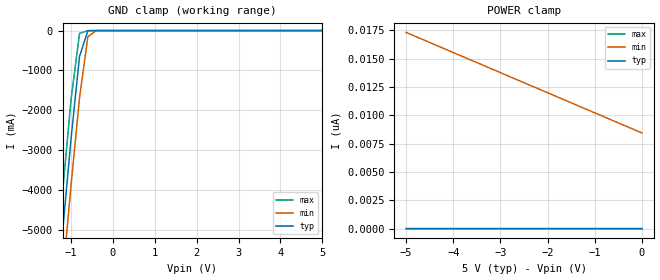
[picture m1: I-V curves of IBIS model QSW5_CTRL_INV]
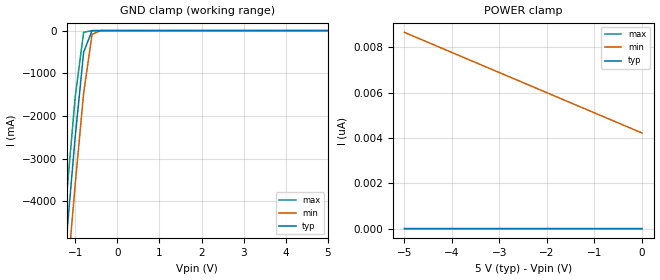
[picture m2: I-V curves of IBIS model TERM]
| I/O Buffer Information Specification (IBIS) Version 3.2 (August 20, 1999)
| IBIS is a standard for electronic behavioral specifications of integrated
| circuit input/output analog characteristics.
[IBIS Ver]   3.2
[File Name]   qs3384.ibs
[File Rev]   2.0
[Date]   Wednesday, June 9, 2004
[Source]   Integrated Device Technology, Inc.
[Notes]   1.Temperatures: typ=25C, min=-40C, max=100C
[Disclaimer]
Integrated Device Technology, Inc. ("IDT") hereby grants the user of this
IBIS model ("User") a non-exclusive, nontransferable license to use this
IBIS model under the following terms: The User is granted this license only
to use the IBIS model for demonstration purposes only and is not granted
rights to sell, copy (except as needed to run the IBIS model), rent, lease
or sub-license (except for demonstration) the IBIS model in whole or in
part, or in modified form to anyone. The User may modify the IBIS model to
suit its specific applications, but  rights to derivative works and such
modifications shall belong to IDT.
THIS IBIS MODEL IS PROVIDED ON AN AS IS" BASIS AND IDT  MAKES ABSOLUTELY NO
WARRANTY WITH RESPECT TO THE INFORMATION CONTAINED HEREIN.  IDT DISCLAIMS
AND USER WAIVES ALL WARRANTIES, EXPRESS AND IMPLIED, INCLUDING WARRANTIES OF
MERCHANTABILITY AND FITNESS FOR A PARTICULAR PURPOSE.  THE ENTIRE RISK AS TO
QUALITY AND PERFORMANCE IS WITH THE USER  ACCORDINGLY, IN NO EVENT SHALL IDT
BE LIABLE FOR ANY DIRECT OR INDIRECT DAMAGES, WHETHER IN CONTRACT OR TORT,
INCLUDING ANY LOST PROFITS OR OTHER INCIDENTAL, CONSEQUENTIAL, EXEMPLARY, OR
PUNITIVE DAMAGES ARISING OUT OF THE USE OR APPLICATION OF THE  IBIS MODEL,
WHETHER OR NOT IDT HAD NOTICE OF SUCH DAMAGES.
IDT reserves the right to make changes without notice to any product herein
to improve reliability, function, or design. IDT does not convey any license
under patent rights or any other intellectual property rights, including
those of third parties. IDT is not obligated to provide maintenance or
support for the licensed IBIS model.
This model is for High-Speed CMOS 10-Bit Bus Switch.
[Copyright]
Copyright 2002, Integrated Device Technology, Inc. All rights reserved.
|   Component QS3384
[Component]   QS3384
[Manufacturer]   Integrated Device Technology
[Package]
|Following package parameters are for TSSOP 24 lead package
| variable   typ   min   max
R_pkg   2.50000m   2.44000m   3.00000m
L_pkg   1.00000nH   0.91000nH   1.74000nH
C_pkg   0.17000pF   0.16000pF   0.27000pF
[Pin]  signal_name   model_name   R_pin   L_pin   C_pin
1   _BEA_   QSW5_CTRL_INV
2   B0   TERM
3   A0   TERM
4   A1   TERM
5   B1   TERM
6   B2   TERM
7   A2   TERM
8   A3   TERM
9   B3   TERM
10   B4   TERM
11   A4   TERM
12   GND   GND
13   _BEB_   QSW5_CTRL_INV
14   A5   TERM
15   B5   TERM
16   B6   TERM
17   A6   TERM
18   A7   TERM
19   B7   TERM
20   B8   TERM
21   A8   TERM
22   A9   TERM
23   B9   TERM
24   VCC   POWER
[Series Switch Groups]
|Function Group States
On A /
On B /
On A B /
Off A B /
[Series Pin Mapping]   pin_2   model_name   function_table_group
3   2   QSW5_SW   A
4   5   QSW5_SW   A
7   6   QSW5_SW   A
8   9   QSW5_SW   A
11   10   QSW5_SW   A
14   15   QSW5_SW   B
17   16   QSW5_SW   B
18   19   QSW5_SW   B
21   20   QSW5_SW   B
22   23   QSW5_SW   B
|   Model QSW5_SW
[Model]   QSW5_SW
Model_type   Series_switch
C_comp   0.0pF   0.0pF   0.0pf
[Temperature Range]   25.00   100.00   -40.00
[Voltage Range]   5.00V   4.75V   5.25V
[On]
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[Off]
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| Models and submodels in the file (3): QSW5_CTRL_INV (Input), TERM (Terminator), QSW5_SW (Series_switch)
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|   Model QSW5_CTRL_INV
[Model]   QSW5_CTRL_INV
Model_type   Input
Vinl =  0.80000V
Vinh =  2.00000V
C_comp   4.20000pF   4.20000pF   4.20000pF
[Temperature Range]   25.00000   100.00000   -40.00000
[Voltage Range]   5.00000V   4.75000V   5.25000V
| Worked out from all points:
|   GND clamp passes 1 mA (typ) near -0.48 V on its own axis
[GND_clamp]
| voltage   I(typ)   I(min)   I(max)
-5V       -51.74A    -52.8A     -50.85A
-1.4V     -7.368A    -8.538A    -6.375A
-1.2V     -4.993A    -6.169A    -3.993A
-1V       -2.692A    -3.858A    -1.708A
-800mV    -650.1mA   -1.689A    -70.61mA
-600mV    -2.541mA   -153.7mA   -3.31mA
-400mV    -3.914uA   -449.3uA   -30.03uA
5V        2.373pA    8.883nA    568.4fA
[POWER_clamp]
| voltage   I(typ)   I(min)   I(max)
-5V       3.268pA    17.31nA    739fA
-3.9V     3.055pA    15.35nA    710.5fA
-3.5V     2.998pA    14.65nA    682.1fA
0V        2.373pA    8.439nA    568.4fA
|   Model TERM
[Model]   TERM
Model_type   Terminator
Vinl =  0.80000V
Vinh =  2.00000V
C_comp   5.70000pF   5.70000pF   5.70000pF
[Temperature Range]   25.00000   100.00000   -40.00000
[Voltage Range]   5.00000V   4.75000V   5.25000V
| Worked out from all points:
|   GND clamp passes 1 mA (typ) near -0.55 V on its own axis
[GND_clamp]
| voltage   I(typ)   I(min)   I(max)
-5V       -51.52A    -52.53A    -50.68A
-1.4V     -7.155A    -8.273A    -6.207A
-1.2V     -4.784A    -5.908A    -3.829A
-1V       -2.494A    -3.606A    -1.556A
-800mV    -507mA     -1.468A    -40.58mA
-600mV    -1.329mA   -90.06mA   -2.011mA
-400mV    -2.283uA   -225uA     -18.42uA
5V        1.357pA    4.443nA    334fA
[POWER_clamp]
| voltage   I(typ)   I(min)   I(max)
-5V       1.805pA    8.655nA    397.9fA
-4.8V     1.776pA    8.477nA    426.3fA
-600mV    1.407pA    4.753nA    355.3fA
0V        1.357pA    4.222nA    326.8fA
